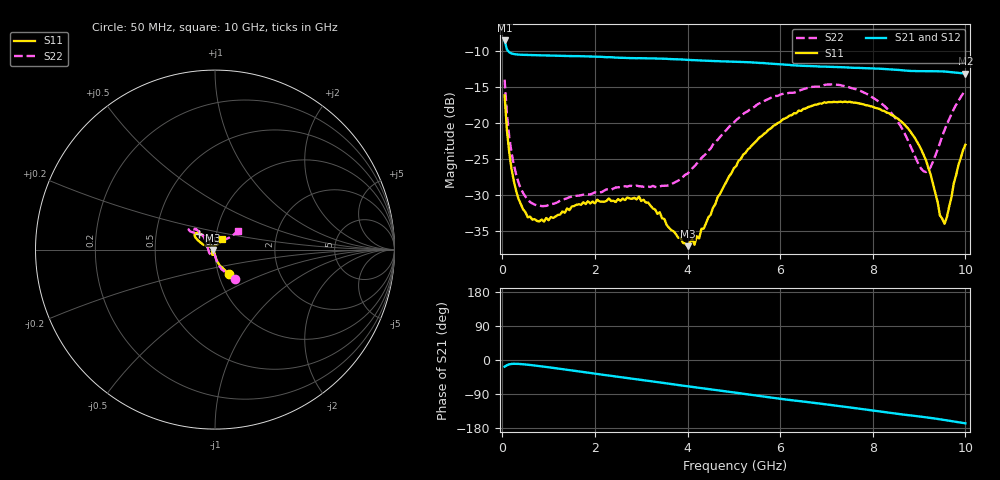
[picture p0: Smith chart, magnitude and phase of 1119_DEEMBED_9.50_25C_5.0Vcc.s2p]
!Hittite Microwave Corp.
!Digital Attenuator/PhaseShifter Rev 1.4.0
!Filename: C:\DATA\DATA\1119_DEEMBED_9.50_25C_5.0Vcc.s2p
!VNA ID: Agilent Technologies,N5224A,MY51441122,A.10.45.03
!Device type:
!2 Port Calibration.
!Temp(C): 25
!Lot Number:
!Serial Number:
!Operator:
!Misc:
!Attenuator:  9.500
# GHZ S DB R 50.0
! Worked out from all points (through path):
!   200 points, 50 MHz to 10 GHz, reference 50 ohm
!   highest |S21| = -8.58 dB at 50 MHz (marker M1); lowest = -13.2 dB at 10 GHz (marker M2)
!   group delay of S21, straight-line fit = 44.8 ps
!   lowest |S11| = -37.1 dB at 4 GHz (marker M3), VSWR 1.03, Z = 48.6 - j0.189 ohm
!   |S11| at or under -10 dB: start of sweep to end of sweep
!   |S22| runs from -31.5 to -14.0 dB; largest |S21 - S12| = 0.00098
!   S11 on the Smith chart (normalised r, x): 50 MHz: 1.12, -0.31; 6.5 GHz: 0.83, +0.15; 10 GHz: 1.08, +0.12
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0.05  -16.19 -60.5  -8.58 -17.6  -8.58 -17.6  -14.01 -56.5
0.15  -24.09 -80.4  -10.22 -11.4  -10.22 -11.4  -21.90 -78.3
0.25  -28.04 -85.9  -10.46 -10.0  -10.47 -10.0  -25.83 -84.6
0.55  -33.06 -95.0  -10.60 -12.4  -10.60 -12.4  -30.62 -91.8
0.9  -33.67 -101.7  -10.65 -17.6  -10.65 -17.6  -31.51 -97.3
1.75  -30.99 -115.0  -10.77 -31.6  -10.78 -31.7  -29.92 -110.0
2.95  -30.20 -116.8  -11.03 -51.5  -11.04 -51.5  -28.76 -147.7
3.4  -32.36 -129.2  -11.09 -59.1  -11.10 -59.2  -28.80 -168.2
4  -37.06 -172.0  -11.27 -69.3  -11.28 -69.4  -27.02 159.4
4.25  -35.98 158.9  -11.35 -73.5  -11.36 -73.6  -25.35 147.8
5.05  -25.98 128.5  -11.53 -86.4  -11.55 -86.5  -19.62 130.3
5.55  -22.02 129.1  -11.69 -94.9  -11.70 -94.9  -17.28 131.2
6.5  -18.06 134.4  -12.09 -109.6  -12.10 -109.6  -15.32 138.7
6.7  -17.60 136.3  -12.13 -112.7  -12.14 -112.7  -15.00 139.8
7.65  -17.22 145.5  -12.37 -127.5  -12.38 -127.5  -15.35 143.8
8.35  -18.65 150.1  -12.57 -139.0  -12.57 -139.0  -18.26 134.4
8.75  -20.68 153.8  -12.78 -145.3  -12.78 -145.3  -22.27 121.0
9.1  -24.46 157.5  -12.83 -150.4  -12.84 -150.4  -26.70 90.8
9.25  -27.15 155.9  -12.83 -152.8  -12.85 -152.9  -26.08 68.8
9.45  -32.79 133.3  -12.85 -156.4  -12.87 -156.5  -22.78 47.6
9.55  -33.96 101.5  -12.88 -158.4  -12.90 -158.4  -20.98 42.6
10  -23.02 53.8  -13.16 -167.1  -13.16 -167.1  -15.49 39.2
